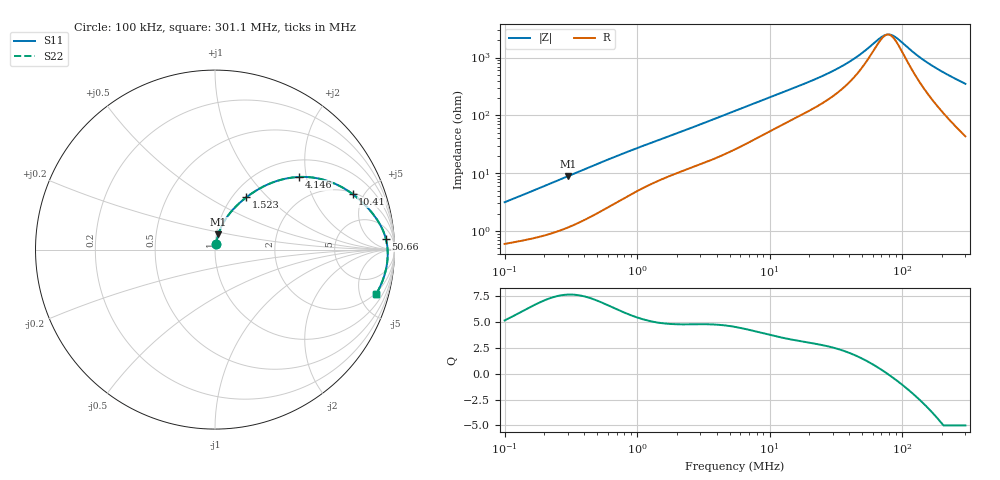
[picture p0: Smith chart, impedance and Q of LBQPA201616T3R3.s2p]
! LBQPA201616T3R3  S-PARAMETER MODEL  ( General Type )
! Model Generated by TAIYO YUDEN Corporation (http://www.ty-top.com)
! Version 1.0
! TAIYO YUDEN Control No. 191025NI43SB-FBB
! Copyright(c) 2019 TAIYO YUDEN CO.,LTD. All Rights Reserved.
! Product Description (link to TY-COMPAS)
! https://ds.yuden.co.jp/TYCOMPAS/or/detail?pn=LBQPA201616T3R3M&u=M
! Products Name : Inductors
! Characteristics :
!  Inductance : 3.3 uH , SRF(min) : 55 MHz , DC Resistance(max) : 0.351 Ohm
!  Rated Current : Saturation :600 mA , Temp Rise : 535 mA (20 degC)
!  Case Size : 2.0 x 1.6 / 0.079 x 0.063 [mm/inch] , Thickness : 1.6 / 0.063 [mm/inch]
!  (Conditions: Temperature = 25 degC , DC Bias Current/Voltage = 0A / 0V)
! External Node Assignments :
!  1  o---GGG---o  2
! GND o---------o GND
! Frequency Range : 0.1MHz  -  301.082333MHz  [ 402 STEP ]
# MHz S RI R 50
! Freq[MHz].  S11 Real  S11 Imag  S21 Real  S21 Imag  S12 Real  S12 Imag  S22 Real  S22 Imag
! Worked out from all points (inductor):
!   401 points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, 100 kHz to 301.1 MHz, reference 50 ohm
!   read as one part in series: L = 4.83 uH near 104.1 kHz
!   highest Q = 7.67 at 300.8 kHz (marker M1), where L = 4.66 uH
!   self-resonance near 77.77 MHz
!   S11 on the Smith chart (normalised r, x): 100 kHz: 1.01, +0.06; 1.523 MHz: 1.16, +0.76; 4.146 MHz: 1.38, +1.82; 10.41 MHz: 2.11, +4.12; 50.66 MHz: 15, +20; 301.1 MHz: 1.87, -6.98
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0.1  0.00687 0.0305  0.9931 -0.0305  0.9931 -0.0305  0.00687 0.0305
0.300829  0.0188 0.0855  0.9812 -0.0855  0.9812 -0.0855  0.0188 0.0855
0.382543  0.0261 0.1065  0.9739 -0.1065  0.9739 -0.1065  0.0261 0.1065
0.771018  0.0732 0.1903  0.9268 -0.1903  0.9268 -0.1903  0.0732 0.1903
1.463388  0.1676 0.2858  0.8324 -0.2858  0.8324 -0.2858  0.1676 0.2858
1.523186  0.1755 0.292  0.8245 -0.292  0.8245 -0.292  0.1755 0.292
2.463055  0.2932 0.3627  0.7068 -0.3627  0.7068 -0.3627  0.2932 0.3627
4.145612  0.4706 0.4048  0.5294 -0.4048  0.5294 -0.4048  0.4706 0.4048
5.487097  0.5747 0.3965  0.4253 -0.3965  0.4253 -0.3965  0.5747 0.3965
7.559447  0.6817 0.3608  0.3183 -0.3608  0.3183 -0.3608  0.6817 0.3608
10.41448  0.7663 0.3097  0.2337 -0.3097  0.2337 -0.3097  0.7663 0.3097
20.99048  0.8841 0.1932  0.1159 -0.1932  0.1159 -0.1932  0.8841 0.1932
34.62902  0.9316 0.1163  0.0684 -0.1163  0.0684 -0.1163  0.9316 0.1163
50.66147  0.9518 0.0607  0.0482 -0.0607  0.0482 -0.0607  0.9518 0.0607
69.79514  0.9603 0.0153  0.0397 -0.0153  0.0397 -0.0153  0.9603 0.0153
75.61571  0.9614 0.00399  0.0386 -0.00399  0.0386 -0.00399  0.9614 0.00399
80.29753  0.9619 -0.00456  0.0381 0.00456  0.0381 0.00456  0.9619 -0.00456
90.54875  0.9624 -0.0219  0.0376 0.0219  0.0376 0.0219  0.9624 -0.0219
127.2702  0.959 -0.0737  0.041 0.0737  0.041 0.0737  0.959 -0.0737
165.114  0.9508 -0.1181  0.0492 0.1181  0.0492 0.1181  0.9508 -0.1181
222.9639  0.9324 -0.1769  0.0676 0.1769  0.0676 0.1769  0.9324 -0.1769
301.0823  0.8993 -0.2451  0.1007 0.2451  0.1007 0.2451  0.8993 -0.2451
